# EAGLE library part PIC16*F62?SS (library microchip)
FLASH-Based 8-Bit CMOS Microcontroller Source: http://ww1.microchip.com/downloads/en/DeviceDoc/40300C.pdf
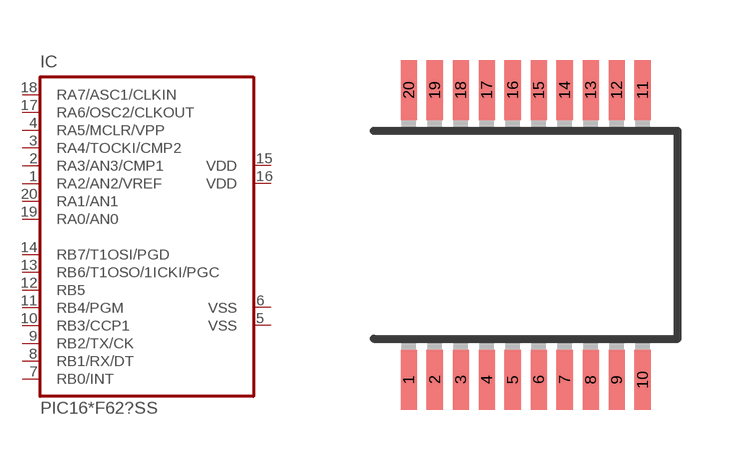
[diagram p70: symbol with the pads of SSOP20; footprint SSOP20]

Designator prefix IC

## PIC16F627SS (MPN: PIC16F627-04I/SS; OC_FARNELL: 9760300; OC_NEWARK: 97K7324), PIC16LF627SS (MF: MICROCHIP; MPN: PIC16LF627-04/SS; OC_FARNELL: unknown; OC_NEWARK: 88K1158)  [SSOP20]
1  RA2/AN2/VREF
2  RA3/AN3/CMP1
3  RA4/TOCKI/CMP2
4  RA5/MCLR/VPP  in
5  VSS  pwr
6  VSS  pwr
7  RB0/INT
8  RB1/RX/DT
9  RB2/TX/CK
10  RB3/CCP1
11  RB4/PGM
12  RB5
13  RB6/T1OSO/1ICKI/PGC
14  RB7/T1OSI/PGD
15  VDD  pwr
16  VDD  pwr
17  RA6/OSC2/CLKOUT
18  RA7/ASC1/CLKIN
19  RA0/AN0
20  RA1/AN1

## PIC16F628SS (MF: MICROCHIP; MPN: PIC16F628-20/SS; OC_FARNELL: 9760440; OC_NEWARK: 23C4984)  [SSOP20]
Pads as for SSOP20

## Footprint SSOP20 (pad centres in mm)
Shrink Small Outline Package package type SS
smd 0.4 x 1.5: 1 -2.925,-3.625; 2 -2.275,-3.625; 3 -1.625,-3.625; 4 -0.975,-3.625; 5 -0.325,-3.625; 6 0.325,-3.625; 7 0.975,-3.625; 8 1.625,-3.625; 9 2.275,-3.625; 10 2.925,-3.625; 11 2.925,3.625; 12 2.275,3.625; 13 1.625,3.625; 14 0.975,3.625; 15 0.325,3.625; 16 -0.325,3.625; 17 -0.975,3.625; 18 -1.625,3.625; 19 -2.275,3.625; 20 -2.925,3.625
